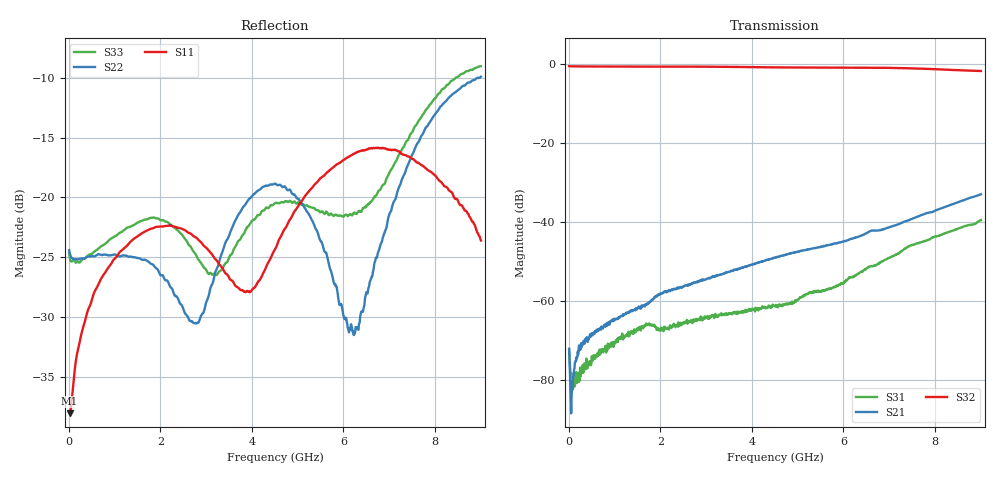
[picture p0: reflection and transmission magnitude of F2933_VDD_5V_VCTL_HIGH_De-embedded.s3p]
! Integrated Device Technology
! Corporate Headquarters
! 6024 Silver Creek Valley Road
! San Jose, CA 95138  USA
! Phone:  1-408-284-8200
! Toll Free:  1-800-223-1366
! Webpage:  http://www.idt.com/
! Timing and RF Division
! 515 Groton Road, Suite 102
! Westford, MA 01886-6024
! Device:  F2933
! Description: 50 Ohm SP2T RF Switch
! Frequency:  50 MHz to 8 GHz
! Package:  4 mm x 4 mm QFN Plastic Package: 16-pin
! Ports:  3 RF, 2 DC
!  Pin  1  = VDD
!  Pin  2  = VCTL
!  Pin  3  = RFC  = Port 3
!  Pin  4  = GND
!  Pin  5  = GND
!  Pin  6  = GND
!  Pin  7  = GND
!  Pin  8  = GND
!  Pin  9  = RF2	= Port 2
!  Pin  10  = GND
!  Pin  11  = GND
!  Pin  12  = RF1	= Port 1
!  Pin  13  = GND
!  Pin  14  = GND
!  Pin  15  = GND
!  Pin  16  = GND
!  EP  = GND
! State:  RF2 selected
! EVKIT Voltages:		VDD  = +5.0 V
!  VCTL = +3.3 V (Logic HIGH)
! Data:  The device was measured on the F2932 EVKit
!  using a calibrated network analyzer with the following
!  EVKIT modifications:
!  R1 = 5.1k ohm
!  C4 = 10 pF
!  These modifications improve the high frequency performance since
!  the standard EVKIT layout has some RF coupling between RFC (pin 3)
!  and VCTL (pin 2).
!  The evaluation board was de-embedded using Automatic Fixture Removal (AFR).
!  The reference plane is the edge of the package pin.
! Misc:
! Date Measured:  2018-5-16
! Date:  2018-5-16
! Note:
!  Integrated Device Technology supplies this data as a sample
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# hz S db R 50
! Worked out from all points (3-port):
!   1000 points, 10 MHz to 9 GHz, reference 50 ohm
!   strongest paths, dB at 10 MHz, 2.26 GHz, 4.509 GHz, 6.759 GHz, 9 GHz:
!     S32: -0.7, -0.8, -1.0, -1.1, -1.9
!     S21: -72.1, -57.0, -49.0, -42.2, -33.0
!     S31: -72.4, -66.4, -61.3, -50.6, -39.6
!   lowest |S11| = -38.1 dB at 19 MHz (marker M1), VSWR 1.03, Z = 51.3 + j0.123 ohm
!   |S11| at or under -10 dB: start of sweep to end of sweep
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1e7  -38.02 0.1  -71.95 -8.5  -72.12 -9.8
     -72.09 -0.5  -24.42 -2.1  -0.67 -0.3
     -72.38 -13.5  -0.67 -0.3  -24.63 -1.9
1.8999e7  -38.07 5.5  -75.29 -29.0  -74.33 -47.5
          -74.69 -28.9  -24.58 -2.3  -0.68 -0.5
          -74.31 -44.6  -0.68 -0.5  -24.91 -2.6
1.35986e8  -34.33 40.0  -75.81 56.8  -80.82 -124.5
           -75.58 63.5  -25.20 3.7  -0.72 -2.6
           -81.52 -133.6  -0.73 -2.6  -25.33 0.5
3.60961e8  -30.28 51.0  -70.05 58.6  -76.91 168.5
           -69.57 49.3  -25.09 9.7  -0.74 -6.6
           -77.25 171.8  -0.74 -6.6  -25.09 5.6
1.413844e9  -23.50 73.6  -62.50 78.9  -68.20 92.2
            -62.47 81.2  -25.02 26.9  -0.77 -25.4
            -67.50 94.8  -0.78 -25.4  -22.33 3.2
2.79969e9  -23.43 79.3  -55.21 90.1  -65.24 50.1
           -55.15 90.2  -30.52 -39.4  -0.79 -50.5
           -64.77 51.5  -0.79 -50.5  -24.99 -45.4
4.5095e9  -24.32 -4.0  -49.04 93.3  -61.13 -40.5
          -49.02 93.1  -18.85 -125.3  -0.97 -82.3
          -61.32 -43.2  -0.98 -82.3  -20.47 -160.2
6.237307e9  -16.32 -17.5  -44.10 95.9  -53.84 -129.4
            -44.08 95.0  -31.29 153.0  -1.02 -114.5
            -53.66 -130.3  -1.02 -114.6  -21.29 -160.7
7.587157e9  -17.03 -15.9  -38.83 95.3  -45.58 -169.7
            -38.83 95.4  -15.67 100.1  -1.27 -141.4
            -45.56 -170.3  -1.27 -141.5  -13.96 152.3
9e9  -23.61 -34.6  -33.05 84.2  -39.60 164.3
     -33.04 84.1  -9.91 78.3  -1.89 -168.5
     -39.56 164.1  -1.90 -168.6  -9.03 123.2
